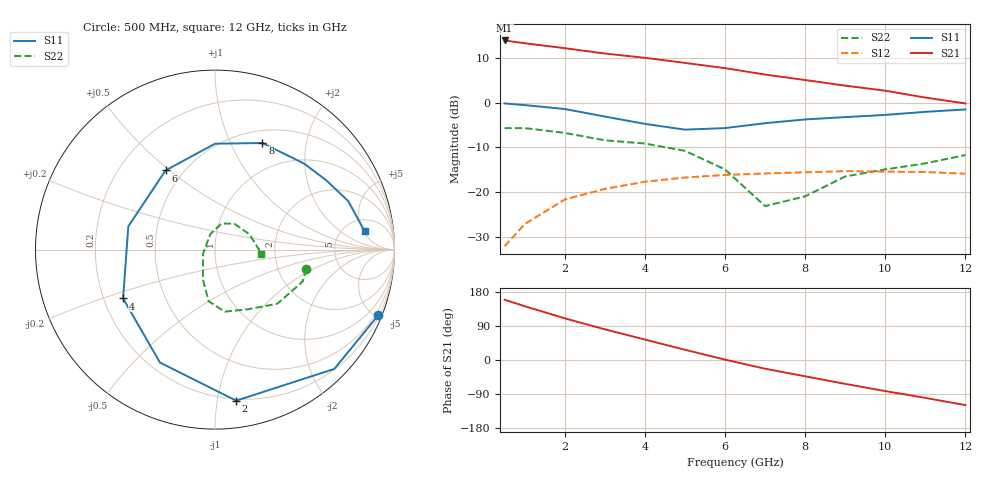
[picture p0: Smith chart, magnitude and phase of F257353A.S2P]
!ATF-25735
!S-PARAMETERS at Vds=3V  Id=20mA.  LAST UPDATED 07-22-92
# ghz s ma r 50
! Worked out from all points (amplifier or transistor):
!   13 points, 500 MHz to 12 GHz, reference 50 ohm
!   highest |S21| = 13.9 dB at 500 MHz (marker M1)
!   |S21| within 3 dB of that: start of sweep to 3.092 GHz
!   unconditionally stable (mu >= 1): 5.524 GHz to end of sweep
!   at 2 GHz: K = 0.44, MSG = 16.9 dB, |S12| = -21.6 dB
!   at 6 GHz: K = 1.04, MAG = 10.7 dB, |S12| = -16.1 dB
!   at 12 GHz: K = 1.13, MAG = 5.7 dB, |S12| = -15.9 dB
!   S11 on the Smith chart (normalised r, x): 500 MHz: 0.28, -5.13; 2 GHz: 0.19, -1.13; 4 GHz: 0.28, -0.23; 6 GHz: 0.40, +0.48; 8 GHz: 0.65, +1.33; 12 GHz: 7.72, +5.37
0.5  0.98 -22.0  4.95 159.0  0.025 77.0  0.52 -12.0
1  0.94 -45.0  4.61 142.0  0.044 64.0  0.52 -20.0
2  0.85 -82.0  4.06 110.0  0.083 45.0  0.46 -41.0
3  0.7 -116.0  3.54 81.0  0.109 24.0  0.38 -61.0
4  0.58 -152.0  3.17 54.0  0.131 12.0  0.35 -81.0
5  0.5 165.0  2.78 27.0  0.146 -7.0  0.29 -97.0
6  0.52 122.0  2.43 1.0  0.156 -20.0  0.18 -112.0
7  0.59 90.0  2.06 -23.0  0.162 -34.0  0.07 -161.0
8  0.65 66.0  1.79 -43.0  0.167 -46.0  0.09 107.0
9  0.69 44.0  1.55 -63.0  0.172 -53.0  0.15 76.0
10  0.73 32.0  1.36 -82.0  0.17 -65.0  0.18 53.0
11  0.79 20.0  1.14 -100.0  0.168 -78.0  0.21 24.0
12  0.84 7.0  0.98 -119.0  0.161 -93.0  0.26 -5.0
